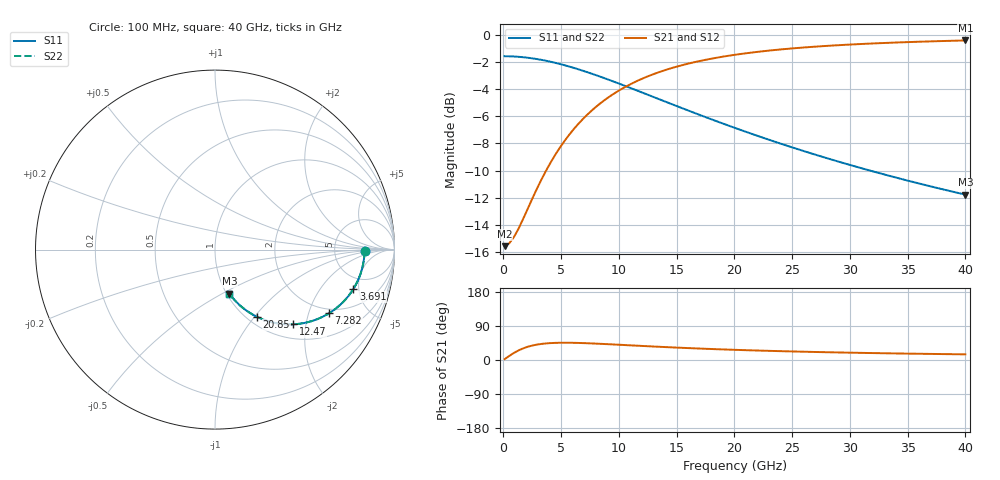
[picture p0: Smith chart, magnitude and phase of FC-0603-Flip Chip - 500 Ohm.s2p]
!Vishay Thin-Film
!FC Family
!Case Size 0603
!Assembly Style Flip Chip
!11/9/2015
!thinfilm@vishay.com
# GHz S MA R 50
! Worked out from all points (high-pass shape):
!   101 points, 100 MHz to 40 GHz, reference 50 ohm
!   highest |S21| = -0.42 dB at 40 GHz (marker M1); lowest = -15.6 dB at 100 MHz (marker M2)
!   |S21| within 3 dB of the highest: 11.52 GHz to end of sweep
!   lowest |S11| = -11.8 dB at 40 GHz (marker M3), VSWR 1.70, Z = 51.5 - j27.1 ohm
!   |S11| at or under -10 dB: 31.76 GHz to end of sweep
!   |S22| runs from -11.8 to -1.6 dB; largest |S21 - S12| = 0
!   S11 on the Smith chart (normalised r, x): 100 MHz: 11, -0; 3.691 GHz: 3.57, -4.37; 7.282 GHz: 1.82, -2.74; 12.47 GHz: 1.29, -1.69; 20.85 GHz: 1.11, -1.03; 40 GHz: 1.03, -0.54
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0.1  0.8333 -0.4  0.1668 2.2  0.1668 2.2  0.8333 -0.4
0.499  0.8327 -2.2  0.1709 10.7  0.1709 10.7  0.8327 -2.2
0.898  0.8314 -3.9  0.1799 18.5  0.1799 18.5  0.8314 -3.9
1.297  0.8292 -5.7  0.1932 25.2  0.1932 25.2  0.8292 -5.7
2.095  0.8228 -9.1  0.2287 34.8  0.2287 34.8  0.8228 -9.1
3.691  0.8018 -15.8  0.3163 43.7  0.3163 43.7  0.8018 -15.8
4.489  0.7879 -19.0  0.3619 45.2  0.3619 45.2  0.7879 -19.0
5.287  0.7722 -22.1  0.4065 45.6  0.4065 45.6  0.7722 -22.1
6.883  0.7368 -27.8  0.4898 44.6  0.4898 44.6  0.7368 -27.8
7.282  0.7274 -29.2  0.5091 44.2  0.5091 44.2  0.7274 -29.2
8.479  0.6984 -33.1  0.5631 42.6  0.5631 42.6  0.6984 -33.1
9.676  0.669 -36.6  0.6111 40.8  0.6111 40.8  0.669 -36.6
10.873  0.6398 -39.8  0.6534 38.9  0.6534 38.9  0.6398 -39.8
12.469  0.602 -43.7  0.7019 36.4  0.7019 36.4  0.602 -43.7
13.666  0.575 -46.4  0.7329 34.6  0.7329 34.6  0.575 -46.4
16.858  0.5096 -52.3  0.7978 30.4  0.7978 30.4  0.5096 -52.3
20.05  0.4541 -57.0  0.8435 26.8  0.8435 26.8  0.4541 -57.0
20.848  0.4416 -58.0  0.8526 26.1  0.8526 26.1  0.4416 -58.0
23.641  0.4022 -61.1  0.8795 23.6  0.8795 23.6  0.4022 -61.1
26.833  0.364 -64.1  0.9025 21.3  0.9025 21.3  0.364 -64.1
33.616  0.3011 -68.8  0.9344 17.5  0.9344 17.5  0.3011 -68.8
40  0.2581 -72.0  0.9523 14.9  0.9523 14.9  0.2581 -72.0
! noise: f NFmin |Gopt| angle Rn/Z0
0.1  9.133e-07  1  4.473e-17  9.979
4.489  9.643e-16  1  0  1.896
8.878  5.165e-08  1  4.192e-15  0.5643
13.27  2.387e-08  1  2.916e-15  0.2608
17.66  0  1  -1.219e-14  0.1489
22.05  0  1  -5.533e-15  0.096
26.43  1.061e-08  1  2.566e-14  0.06694
30.82  0  1  -4.728e-15  0.0493
35.21  0  1  -2.382e-14  0.03781
40  5.364e-09  1  4.675e-14  0.0293
